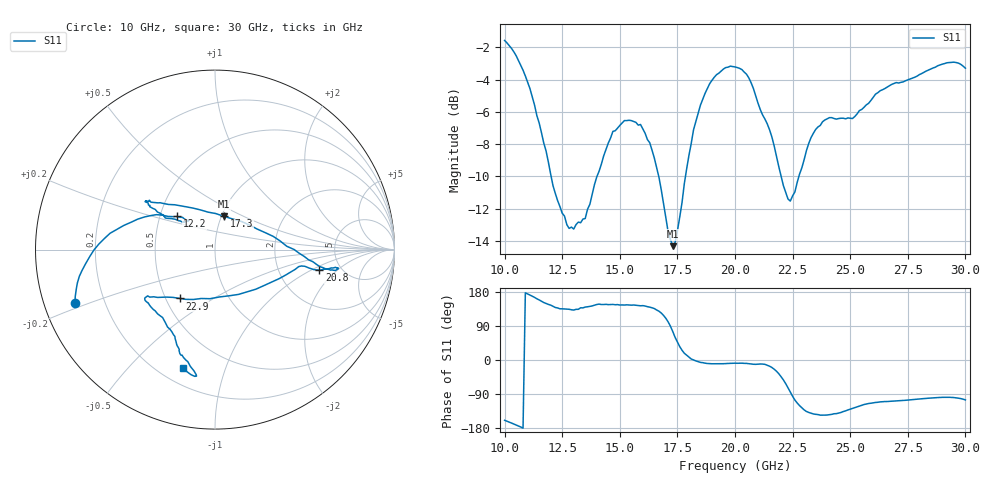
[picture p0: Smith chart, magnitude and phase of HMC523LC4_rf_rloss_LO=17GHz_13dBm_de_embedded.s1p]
!Hittite Microwave Corporation
!20 Alpha Rd
!Chelmsford, MA 01824
!Tel: 978-250-3343
!Fax: 978-250-3373
!Device: HMC523LC4, 10-30 GHz, GaAs MMIC Double-Balanced Mixer
!Misc: RF Return Loss with LO=17GHz at 13 dBm, Room
# MHZ S MA R 50
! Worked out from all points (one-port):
!   201 points, 10 GHz to 30 GHz, reference 50 ohm
!   lowest |S11| = -14.3 dB at 17.3 GHz (marker M1), VSWR 1.48, Z = 51.4 + j19.8 ohm
!   |S11| at or under -10 dB: 12.02 GHz to 14.01 GHz (1.991 GHz wide, 15.3 % of centre); 16.69 GHz to 17.85 GHz (1.161 GHz wide, 6.72 % of centre); 22 GHz to 22.77 GHz (770.5 MHz wide, 3.44 % of centre)
!   S11 on the Smith chart (normalised r, x): 10 GHz: 0.09, -0.18; 12.2 GHz: 0.61, +0.25; 17.3 GHz: 1.03, +0.40; 20.8 GHz: 3.44, -1.22; 22.9 GHz: 0.59, -0.36; 30 GHz: 0.29, -0.72
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10000  0.835 -159.1
10500  0.749 -171.2
11100  0.592 171.2
11600  0.432 155.1
12200  0.28 138.6
12500  0.243 135.1
12800  0.218 133.8
13500  0.234 139.7
14500  0.401 146.1
15000  0.455 145.1
15600  0.468 145.2
16300  0.402 139.5
17300  0.192 74.9
17500  0.214 47.5
18500  0.526 -6.3
19200  0.654 -10.1
20000  0.691 -8.4
20800  0.592 -11.2
21600  0.419 -19.7
22300  0.269 -73.2
22500  0.275 -95.9
22900  0.336 -126.0
23800  0.467 -145.5
25000  0.479 -129.7
26100  0.569 -112.1
27500  0.63 -105.7
29200  0.712 -98.3
30000  0.685 -105.3
